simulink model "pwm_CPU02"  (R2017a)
settings: Solver=FixedStepDiscrete  StartTime=0.0  StopTime=inf  RelTol=1e-3  EnableMultiTasking=on
undefined symbols (not defined in the file): A, Compare, conversion, DCAEVT1, DCAEVT1FILT, Digital, Down, Event, Filtered, GPTRIP1SEL, GPTRIP2SEL, input, Module, of, start, Trip, TZ1, TZ2, Up, version, Zone
libraries: c2837xDlib x1, c2802xlib x1

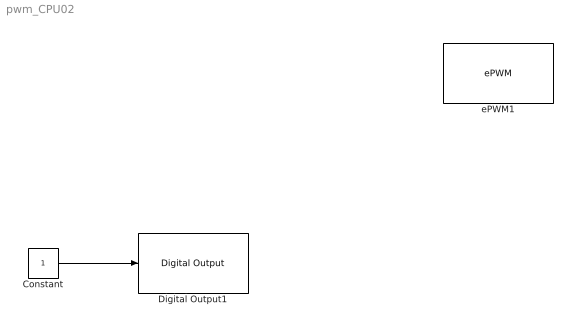
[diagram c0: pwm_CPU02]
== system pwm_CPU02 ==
  Constant : Constant  SampleTime=-1
  Digital Output1 : c2837xDlib/Digital Output  GPIO_Number=GPIO24~GPIO31  GPIO_Bit0=off  GPIO_BIT0_Toggle=off  GPIO_Bit1=off  GPIO_BIT1_Toggle=on  GPIO_Bit2=off  GPIO_BIT2_Toggle=off  GPIO_Bit3=off  GPIO_BIT3_Toggle=off  GPIO_Bit4=off  GPIO_BIT4_Toggle=off  GPIO_Bit5=off  GPIO_BIT5_Toggle=off  GPIO_Bit6=off  GPIO_BIT6_Toggle=off  GPIO_Bit7=on  GPIO_BIT7_Toggle=off
  ePWM1 : c2802xlib/ePWM  useModule=ePWM1  ePWMxLINKTBPRD=Not Linked  periodUnits=Clock cycles  timerSource=Specify via dialog  timerPeriod_clk=2000  timerPeriod_sec=0.00002  tbshadow=Counter equals to zero  countingMode=Up-Down  phaseActiveEnable=Disable  phaseDirection=Count down after sync  phaseActive=0  synchronizationEnable=off  dcaevt1Sync=off  dcbevt1Sync=off  synchronizationOption=Disable  clockPrescale=1  HSclockPrescale=1  enswap=off  ePWMxAStatus=on  ePWMxAactionLogic1=Set  ePWMxAactionLogic2=Clear  ePWMxAactionLogic3=Clear  ePWMxAactionLogic4=Set  ePWMxAactionLogic5=Do nothing  ePWMxAactionLogic6=Do nothing  ePWMxALoadMode=Load on counter equals to zero (CTR=Zero)  ePWMxACSFenable=off  ePWMxACSFvalue=Forcing disable  ePWMxASFreload=Zero  ePWMxBStatus=off  ePWMxBactionLogic1=Set  ePWMxBactionLogic2=Clear  ePWMxBactionLogic3=Do nothing  ePWMxBactionLogic4=Do nothing  ePWMxBactionLogic5=Clear  ePWMxBactionLogic6=Set  ePWMxBLoadMode=Load on counter equals to zero (CTR=Zero)  ePWMxBCSFenable=off  ePWMxBCSFvalue=Forcing disable  ePWMxBSFreload=Zero  ePWNxBOutWay=off  ePWMxLINKCMPA=Not Linked  CMPAUnits=Clock cycles  CMPASource=Specify via dialog  CMPAValue_per=100  CMPAValue_clk=500  enCMPAshadow=Counter equals to zero  ePWMxLINKCMPB=Not Linked  CMPBUnits=Clock cycles  CMPBSource=Specify via dialog  CMPBValue_per=0  CMPBValue_clk=500  enCMPBshadow=Counter equals to zero  ePWMxLINKCMPC=Not Linked  CMPCUnits=Clock cycles  CMPCSource=Specify via dialog  CMPCValue_per=50  CMPCValue_clk=32000  enCMPCshadow=Counter equals to zero  ePWMxLINKCMPD=Not Linked  CMPDUnits=Clock cycles  CMPDSource=Specify via dialog  CMPDValue_per=50  CMPDValue_clk=32000  enCMPDshadow=Counter equals to zero  enableDBePWMxA=on  enableDBePWMxB=on  enhalfcycle=off  DBpolarity=Active high complementary (AHC)  DBedgeDelay=Positive  DBSource_ePWMxA=ePWMxA  DBSource_ePWMxB=ePWMxA  DBperiodSource=Specify via dialog  REDperiod=50  FEDperiod=50  adcstartModuleA=off  adcrequestEventA=First event  adcstartEventA=Digital Compare Module A Event 1 start of conversion (DCAEVT1.soc)  adcstartEventA_type2=Counter equals to zero (CTR=Zero)  adcstartModuleB=off  adcrequestEventB=First event  adcstartEventB=Counter equals to zero (CTR=Zero)  adcstartEventB_type2=Counter equals to zero (CTR=Zero)  intEn=off  intPrd=First event  intSel=Counter equals to zero (CTR=Zero)  intSel_type2=Counter equals to zero (CTR=Zero)  hrpe=on  enHRPWM=on  HRPWM_LoadMode=Counter equals to period (CTR=PRD)  HRPWM_CTLMode=Duty or Period control mode  HRPWM_EDGMode=Both edge  hrpeb=off  enHRPWMB=off  HRPWM_LoadModeB=Counter equals to zero (CTR=ZERO)  HRPWM_CTLModeB=Duty or Period control mode  HRPWM_EDGModeB=Both edge  enSFO=on  enautoconv=on  chopperEnable=off  chopperFrequency=1  chopperFirstwidth=1  chopperDuty=12.5%  tripZonesource=Specify via dialog  tzselOSHT1=off  tzselOSHT2=off  tzselOSHT3=off  tzselOSHDCAEV1=off  tzselOSHDCBEV1=off  tzselCBC1=off  tzselCBC2=off  tzselCBC3=off  tzselCBCDCAEV2=off  tzselCBCDCBEV2=off  tzselOSHT4=off  tzselOSHT5=off  tzselOSHT6=off  tzselCBC4=off  tzselCBC5=off  tzselCBC6=off  enTzOstIntr=off  enTzCbcIntr=off  enTzDCAEVT1Intr=off  enTzDCAEVT2Intr=off  enTzDCBEVT1Intr=off  enTzDCBEVT2Intr=off  ePWMxAforced=No action  ePWMxBforced=No action  DCAEVT1forced=No action  DCBEVT1forced=No action  DCAEVT2forced=No action  DCBEVT2forced=No action  dcah=Trip Zone 1 input (TZ1)  dcal=Trip Zone 2 input (TZ2)  dcbh=Trip Zone 1 input (TZ1)  dcbl=Trip Zone 2 input (TZ2)  dcah_type2=GPTRIP1SEL/(TZ1)  dcal_type2=GPTRIP2SEL/(TZ2)  dcbh_type2=GPTRIP1SEL/(TZ1)  dcbl_type2=GPTRIP2SEL/(TZ2)  gendcaevt1=Event disabled  gendcaevt2=Event disabled  gendcbevt1=Event disabled  gendcbevt2=Event disabled  dcaevt1src=DCAEVT1 with sync  dcaevt2src=DCAEVT2 with sync  dcbevt1src=DCBEVT1 with sync  dcbevt2src=DCBEVT2 with sync  pulsesel=Counter equals to zero (CTR=Zero)  blankinv=off  blankoffset=0  blankwidth=0  evsrcsel=Filtered version of DCAEVT1 (DCAEVT1FILT)  encape=off  PwmType=C2000_Type4
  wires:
  Constant/1 -> Digital Output1/1
